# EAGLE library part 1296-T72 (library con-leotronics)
1.27mm SINGLE ROW FEMALE SOCKET Source: http://www.leotronics.co.uk/Conexcon/Data%20Sheets/sec.%20A/1296ing.pdf
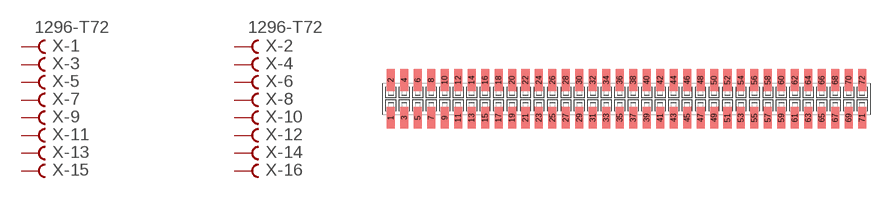
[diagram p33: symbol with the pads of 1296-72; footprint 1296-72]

Designator prefix X; gates -1=FVAL -2=FVAL -3=F -4=F -5=F -6=F -7=F -8=F -9=F -10=F -11=F -12=F -13=F -14=F -15=F -16=F -17=F -18=F -19=F -20=F -21=F -22=F -23=F -24=F -25=F -26=F -27=F -28=F -29=F -30=F -31=F -32=F -33=F -34=F -35=F -36=F -37=F -38=F -39=F -40=F -41=F -42=F -43=F -44=F -45=F -46=F -47=F -48=F -49=F -50=F -51=F -52=F -53=F -54=F -55=F -56=F -57=F -58=F -59=F -60=F -61=F -62=F -63=F -64=F -65=F -66=F -67=F -68=F -69=F -70=F -71=F -72=F

## 1296-T72 (OC_FARNELL: unknown; OC_NEWARK: unknown)  [1296-72]
1  -1:B  pas
2  -2:B  pas
3  -3:B  pas
4  -4:B  pas
5  -5:B  pas
6  -6:B  pas
7  -7:B  pas
8  -8:B  pas
9  -9:B  pas
10  -10:B  pas
11  -11:B  pas
12  -12:B  pas
13  -13:B  pas
14  -14:B  pas
15  -15:B  pas
16  -16:B  pas
17  -17:B  pas
18  -18:B  pas
19  -19:B  pas
20  -20:B  pas
21  -21:B  pas
22  -22:B  pas
23  -23:B  pas
24  -24:B  pas
25  -25:B  pas
26  -26:B  pas
27  -27:B  pas
28  -28:B  pas
29  -29:B  pas
30  -30:B  pas
31  -31:B  pas
32  -32:B  pas
33  -33:B  pas
34  -34:B  pas
35  -35:B  pas
36  -36:B  pas
37  -37:B  pas
38  -38:B  pas
39  -39:B  pas
40  -40:B  pas
41  -41:B  pas
42  -42:B  pas
43  -43:B  pas
44  -44:B  pas
45  -45:B  pas
46  -46:B  pas
47  -47:B  pas
48  -48:B  pas
49  -49:B  pas
50  -50:B  pas
51  -51:B  pas
52  -52:B  pas
53  -53:B  pas
54  -54:B  pas
55  -55:B  pas
56  -56:B  pas
57  -57:B  pas
58  -58:B  pas
59  -59:B  pas
60  -60:B  pas
61  -61:B  pas
62  -62:B  pas
63  -63:B  pas
64  -64:B  pas
65  -65:B  pas
66  -66:B  pas
67  -67:B  pas
68  -68:B  pas
69  -69:B  pas
70  -70:B  pas
71  -71:B  pas
72  -72:B  pas

## Footprint 1296-72 (pad centres in mm)
1.27mm SINGLE ROW FEMALE SOCKET Source: http://www.leotronics.co.uk/Conexcon/Data%20Sheets/sec.%20A/1296ing.pdf
smd 0.76 x 2.05: 1 -22.225,-1.78; 2 -22.225,1.78; 3 -20.955,-1.78; 4 -20.955,1.78; 5 -19.685,-1.78; 6 -19.685,1.78; 7 -18.415,-1.78; 8 -18.415,1.78; 9 -17.145,-1.78; 10 -17.145,1.78; 11 -15.875,-1.78; 12 -15.875,1.78; 13 -14.605,-1.78; 14 -14.605,1.78; 15 -13.335,-1.78; 16 -13.335,1.78; 17 -12.065,-1.78; 18 -12.065,1.78; 19 -10.795,-1.78; 20 -10.795,1.78; 21 -9.525,-1.78; 22 -9.525,1.78; 23 -8.255,-1.78; 24 -8.255,1.78; 25 -6.985,-1.78; 26 -6.985,1.78; 27 -5.715,-1.78; 28 -5.715,1.78; 29 -4.445,-1.78; 30 -4.445,1.78; 31 -3.175,-1.78; 32 -3.175,1.78; 33 -1.905,-1.78; 34 -1.905,1.78; 35 -0.635,-1.78; 36 -0.635,1.78; 37 0.635,-1.78; 38 0.635,1.78; 39 1.905,-1.78; 40 1.905,1.78; 41 3.175,-1.78; 42 3.175,1.78; 43 4.445,-1.78; 44 4.445,1.78; 45 5.715,-1.78; 46 5.715,1.78; 47 6.985,-1.78; 48 6.985,1.78; 49 8.255,-1.78; 50 8.255,1.78; 51 9.525,-1.78; 52 9.525,1.78; 53 10.795,-1.78; 54 10.795,1.78; 55 12.065,-1.78; 56 12.065,1.78; 57 13.335,-1.78; 58 13.335,1.78; 59 14.605,-1.78; 60 14.605,1.78; 61 15.875,-1.78; 62 15.875,1.78; 63 17.145,-1.78; 64 17.145,1.78; 65 18.415,-1.78; 66 18.415,1.78; 67 19.685,-1.78; 68 19.685,1.78; 69 20.955,-1.78; 70 20.955,1.78; 71 22.225,-1.78; 72 22.225,1.78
